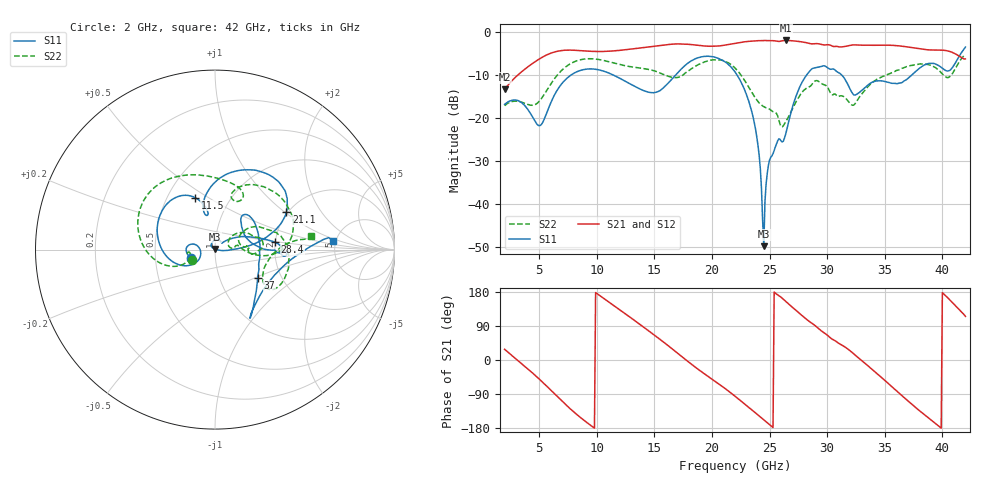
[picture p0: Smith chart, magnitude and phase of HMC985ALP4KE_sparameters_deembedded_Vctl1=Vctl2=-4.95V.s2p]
!s2p File: Measurements: S11, S21, S12, S22
# GHz S dB R 50.0
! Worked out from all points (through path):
!   401 points, 2 GHz to 42 GHz, reference 50 ohm
!   highest |S21| = -2.05 dB at 26.4 GHz (marker M1); lowest = -13.4 dB at 2 GHz (marker M2)
!   lowest |S11| = -49.8 dB at 24.5 GHz (marker M3), VSWR 1.01, Z = 49.9 + j0.308 ohm
!   |S11| at or under -10 dB: start of sweep to 7.811 GHz; 22.16 GHz to 28.24 GHz (6.078 GHz wide, 24.1 % of centre); 31.24 GHz to 37.37 GHz (6.139 GHz wide, 17.9 % of centre)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
!   |S22| runs from -22.1 to -5.3 dB; largest |S21 - S12| = 0.00088
!   S11 on the Smith chart (normalised r, x): 2 GHz: 0.76, -0.07; 11.5 GHz: 0.68, +0.44; 21.1 GHz: 1.97, +1.03; 28.4 GHz: 2.00, +0.18; 37 GHz: 1.52, -0.52; 42 GHz: 4.77, +0.78
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2  -16.88 -161.7  -13.43 28.3  -13.44 28.3  -17.18 -155.5
5  -21.83 -172.4  -6.37 -50.1  -6.37 -50.1  -16.18 -159.7
6.3  -14.85 -150.2  -4.75 -88.3  -4.76 -88.3  -11.02 -161.5
8.7  -8.91 150.4  -4.44 -154.6  -4.44 -154.6  -6.46 151.3
11.5  -10.16 111.1  -4.47 143.2  -4.47 143.2  -7.30 105.1
13.6  -13.11 101.1  -3.85 97.2  -3.86 97.2  -8.40 75.7
15.4  -13.82 105.8  -3.26 56.5  -3.26 56.5  -9.49 62.0
17.9  -7.33 80.3  -2.94 -3.5  -2.94 -3.4  -9.21 72.0
21.1  -6.96 27.6  -3.14 -74.3  -3.14 -74.3  -6.85 16.1
22  -9.34 17.1  -2.71 -95.5  -2.71 -95.5  -8.44 0.6
23.6  -20.19 0.0  -2.17 -135.2  -2.17 -135.1  -14.71 -4.6
24.5  -49.78 107.8  -2.08 -157.8  -2.08 -157.8  -17.41 7.9
25  -29.81 132.6  -2.10 -170.6  -2.10 -170.5  -18.00 10.8
26.4  -23.77 41.5  -2.05 154.7  -2.05 154.8  -20.97 32.6
28.4  -9.43 6.9  -2.71 102.8  -2.71 102.8  -12.86 18.3
28.7  -8.60 2.0  -2.85 96.5  -2.85 96.5  -12.18 16.3
30.7  -8.95 -3.0  -3.44 50.6  -3.44 50.6  -14.51 2.1
32.5  -14.64 31.3  -3.09 11.0  -3.09 11.0  -16.45 27.3
35.4  -11.82 19.4  -3.15 -64.5  -3.15 -64.4  -9.80 19.4
37  -10.88 -33.6  -3.57 -107.6  -3.57 -107.6  -8.06 5.0
39.8  -8.08 -57.6  -4.29 -177.1  -4.28 -177.1  -9.25 -36.1
42  -3.59 4.0  -6.34 115.1  -6.34 115.2  -5.34 8.3
